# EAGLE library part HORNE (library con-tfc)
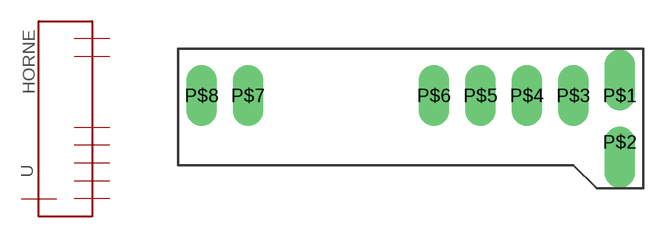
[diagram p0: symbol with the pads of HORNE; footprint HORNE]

Designator prefix -

## HORNE  [HORNE]
P$1  P$1  pas
P$2  P$2  pas
P$3  P$3  pas
P$4  P$4  pas
P$5  P$5  pas
P$6  P$6  pas
P$7  P$7  pas
P$8  P$8  pas

## Footprint HORNE (pad centres in mm)
drill 0.5 pad 1.676 offset: P$1 8.89,1.27; P$2 8.89,-1.27
drill 0.5 pad 1.676 long: P$3 6.35,1.27; P$4 3.81,1.27; P$5 1.27,1.27; P$6 -1.27,1.27; P$7 -11.43,1.27; P$8 -13.97,1.27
